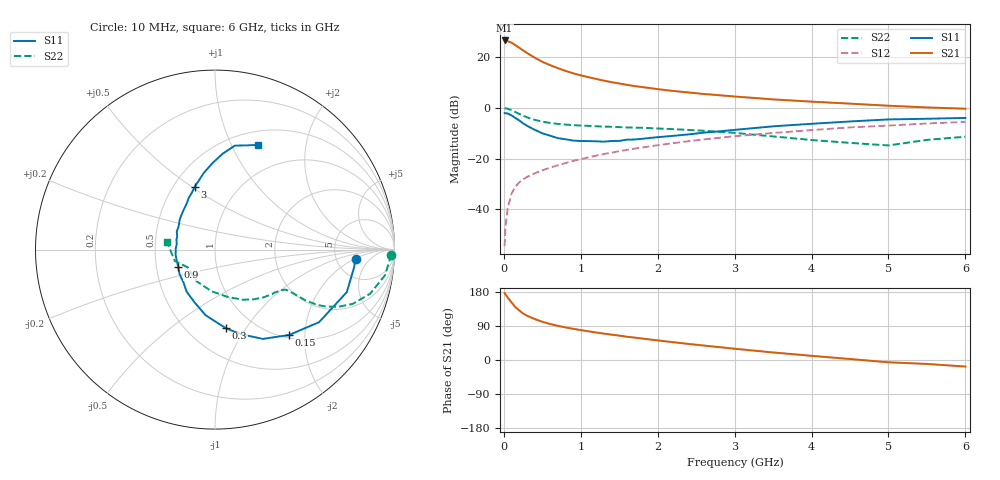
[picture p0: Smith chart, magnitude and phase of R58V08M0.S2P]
! SIEMENS Small Signal Semiconductors
! BFR183
! Si NPN RF Bipolar Junction Transistor in SOT23
! VCE = 8 V  IC = 8 mA
! Common Emitter S-Parameters:  May  1996
# GHz  S  MA  R  50
!  f  S11  S21  S12  S22
! GHz  MAG  ANG  MAG  ANG  MAG  ANG  MAG  ANG
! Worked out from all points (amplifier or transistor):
!   36 points, 10 MHz to 6 GHz, reference 50 ohm
!   highest |S21| = 26.5 dB at 10 MHz (marker M1)
!   |S21| within 3 dB of that: start of sweep to 207.1 MHz
!   unconditionally stable (mu >= 1): 890 MHz to 2.613 GHz
!   at 250 MHz: K = 0.54, MSG = 25.4 dB, |S12| = -28.2 dB
!   at 1.4 GHz: K = 1.05, MAG = 12.5 dB, |S12| = -17.6 dB
!   at 6 GHz: K = 0.88, MSG = 2.6 dB, |S12| = -5.5 dB
!   lowest NFmin = 1.30 dB at 450 MHz
!   S11 on the Smith chart (normalised r, x): 10 MHz: 7.75, -2.04; 150 MHz: 1.05, -1.66; 300 MHz: 0.75, -0.82; 900 MHz: 0.65, -0.13; 3 GHz: 0.64, +0.51; 6 GHz: 0.66, +1.27
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0.01  0.7849 -3.7  21.04 176.6  0.0019 85.7  0.9815 -1.6
0.02  0.7811 -7.3  20.95 173.4  0.0044 83.4  0.9749 -3.5
0.05  0.7715 -17.9  20.4 165.0  0.0105 78.4  0.9578 -8.6
0.1  0.7069 -34.9  19.02 151.7  0.0205 74.1  0.8983 -15.9
0.15  0.6298 -49.1  17.03 139.7  0.028 68.2  0.8249 -21.5
0.2  0.5645 -61.8  15.15 130.7  0.034 64.9  0.7588 -24.8
0.25  0.4949 -72.6  13.45 122.8  0.0391 62.2  0.6978 -27.1
0.3  0.4431 -82.0  11.96 116.8  0.0435 61.6  0.6485 -28.4
0.4  0.3692 -98.2  9.668 108.2  0.0512 61.0  0.5791 -29.3
0.5  0.3151 -111.2  8.016 100.8  0.0588 61.0  0.5342 -29.3
0.6  0.2826 -124.0  6.892 95.1  0.0666 61.7  0.5032 -29.2
0.7  0.2532 -134.0  6.021 90.3  0.0737 62.9  0.4822 -29.2
0.9  0.2265 -154.8  4.76 82.4  0.09 63.0  0.4555 -29.5
1.1  0.2212 -172.5  3.988 75.8  0.1059 63.1  0.4398 -30.9
1.3  0.2154 171.7  3.412 69.7  0.1233 62.8  0.4264 -32.2
1.6  0.236 154.5  2.817 61.4  0.1488 61.7  0.41 -35.6
2.2  0.28 129.1  2.14 47.0  0.2016 57.7  0.3805 -44.3
3  0.3671 108.0  1.664 29.7  0.2756 50.0  0.3207 -60.7
3.5  0.4313 98.4  1.46 19.9  0.3189 44.1  0.2731 -75.1
4.5  0.5377 85.2  1.204 2.6  0.4113 32.4  0.2039 -119.7
5.5  0.6076 72.9  1.014 -10.4  0.4903 20.7  0.2336 -164.5
6  0.6312 67.5  0.958 -17.3  0.528 13.1  0.2696 171.1
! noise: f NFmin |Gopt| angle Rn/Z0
0.45  1.3  0.17  43  0.21
0.9  1.35  0.21  115  0.2
1.8  2.05  0.33  -177  0.14
